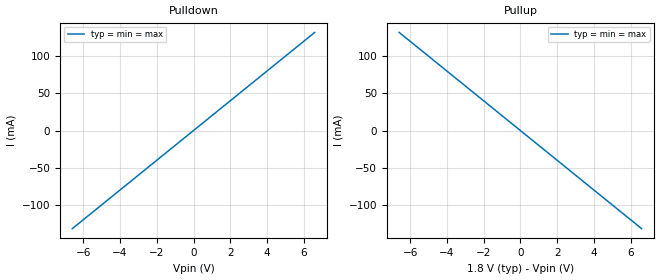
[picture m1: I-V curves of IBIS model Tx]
[IBIS Ver]   5.0
[File Name]   Tx.ibs
[File Rev]   1.0
[Component]   Tx
[Manufacturer] My Company
[Package]
R_pkg  0.0   NA   NA
L_pkg  0.0   NA   NA
C_pkg  0.0   NA   NA
[Pin]   signal_name   model_name   R_pin L_pin  C_pin
1p   Tx_p   Tx
1n   Tx_n   Tx
[Diff_Pin] inv_pin vdiff tdelay_typ tdelay_min tdelay_max
1p   1n   NA   NA   NA   NA
| Models and submodels in the file (1): Tx (Output)
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[Model] Tx
Model_type Output
C_comp 0p 0p 0p
Cref = 0
Vref = 0.5
Rref = 50
Vmeas = 0.5
[Temperature_Range] 25 125 0
[Voltage Range] 1.8 1.8 1.8
[Algorithmic Model]
Executable Windows_cl16.00.30319.01_64 Tx_x64.dll Tx.ami
Executable Windows_cl16.00.30319.01_32 Tx.dll Tx.ami
[End Algorithmic Model]
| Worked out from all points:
|   slope of the pulldown table from 0 to 0.27 V, typ, clamps not added: 50 ohm
|   slope of the pullup table from 0 to 0.27 V, typ, clamps not added: 50 ohm
[Pulldown]
-6.6V     -132mA     -132mA     -132mA
0V        0A         0A         0A
6.6V      132mA      132mA      132mA
[Pullup]
-6.6V     132mA      132mA      132mA
0V        0A         0A         0A
6.6V      -132mA     -132mA     -132mA
[GND Clamp]
-6.6V     0A         0A         0A
0V        0A         0A         0A
6.6V      0A         0A         0A
[Power Clamp]
-6.6V     0A         0A         0A
0V        0A         0A         0A
6.6V      0A         0A         0A
[Ramp]
dV/dt_r 0.4/1.5p 0.4/1.5p 0.4/1.5p
dV/dt_f 0.4/1.5p 0.4/1.5p 0.4/1.5p
